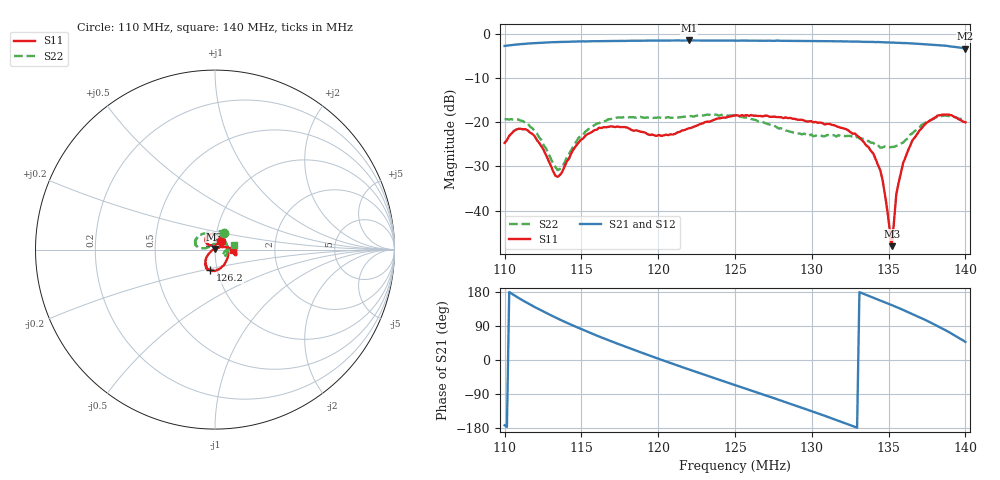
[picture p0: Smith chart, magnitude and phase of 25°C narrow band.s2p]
!Agilent Technologies,E8362C,SG49020144,A.09.33.09
!Agilent E8362C: A.09.33.09
!Date: Friday, October 10, 2025 08:48:52
!Correction: S11(Full 2 Port(1,2))
!S21(Full 2 Port(1,2))
!S12(Full 2 Port(1,2))
!S22(Full 2 Port(1,2))
!S2P File: Measurements: S11, S21, S12, S22:
# Hz S  dB  R 50
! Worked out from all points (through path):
!   201 points, 110 MHz to 140 MHz, reference 50 ohm
!   highest |S21| = -1.50 dB at 122 MHz (marker M1); lowest = -3.3 dB at 140 MHz (marker M2)
!   lowest |S11| = -48.1 dB at 135.2 MHz (marker M3), VSWR 1.01, Z = 49.7 + j0.304 ohm
!   |S11| at or under -10 dB: start of sweep to end of sweep
!   |S22| runs from -30.8 to -18.3 dB; largest |S21 - S12| = 0.0065
!   S11 on the Smith chart (normalised r, x): 110 MHz: 1.06, +0.10; 126.2 MHz: 0.93, -0.22; 140 MHz: 1.22, -0.01
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1.1e8  -24.69 56.2  -2.74 -172.4  -2.73 -172.6  -19.29 60.9
1.1075e8  -21.67 68.6  -2.44 167.7  -2.47 167.6  -19.42 74.1
1.115e8  -21.84 63.3  -2.20 149.9  -2.20 149.8  -20.30 74.2
1.1345e8  -32.39 102.9  -1.85 109.5  -1.87 109.5  -30.84 120.4
1.151e8  -23.71 138.9  -1.69 79.7  -1.72 79.7  -22.87 174.0
1.178e8  -21.11 93.8  -1.61 36.1  -1.61 35.8  -18.78 165.0
1.2005e8  -22.88 26.0  -1.52 2.8  -1.55 2.8  -18.92 162.9
1.22e8  -21.38 -37.5  -1.50 -24.9  -1.50 -24.9  -18.68 160.6
1.25e8  -18.47 -90.3  -1.54 -66.2  -1.53 -66.2  -18.50 139.5
1.262e8  -18.53 -102.6  -1.55 -82.4  -1.57 -82.7  -19.38 122.9
1.28e8  -18.89 -114.2  -1.58 -107.2  -1.56 -107.4  -21.37 87.1
1.301e8  -20.02 -119.8  -1.63 -136.8  -1.62 -136.8  -23.18 29.0
1.328e8  -22.57 -133.3  -1.76 -176.2  -1.78 -176.5  -23.59 -28.8
1.34e8  -27.09 -145.3  -1.83 164.7  -1.85 164.7  -24.69 -37.6
1.346e8  -32.95 -157.4  -1.90 155.0  -1.93 155.0  -25.73 -32.0
1.3505e8  -43.61 166.3  -1.94 147.5  -1.97 147.6  -25.69 -23.6
1.352e8  -48.07 129.3  -1.99 145.0  -1.98 145.0  -25.61 -22.1
1.355e8  -36.39 33.5  -2.02 139.9  -2.03 139.9  -25.37 -14.7
1.3595e8  -29.21 28.1  -2.09 132.1  -2.09 132.0  -24.60 -5.0
1.3655e8  -24.10 11.7  -2.16 121.4  -2.17 121.3  -22.51 0.2
1.382e8  -18.46 -8.8  -2.57 89.2  -2.55 89.3  -18.71 -1.5
1.4e8  -20.02 -1.8  -3.33 47.8  -3.29 47.7  -19.21 14.4
